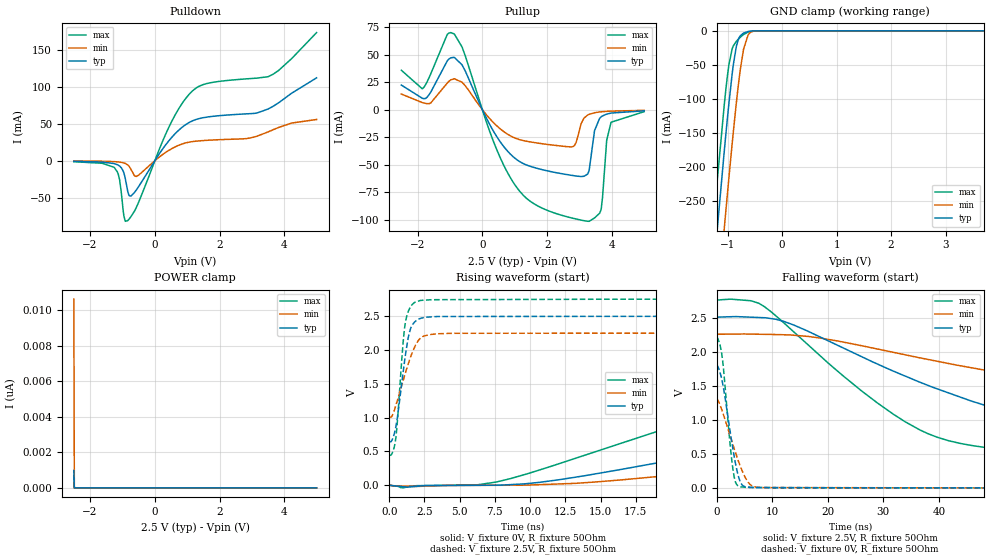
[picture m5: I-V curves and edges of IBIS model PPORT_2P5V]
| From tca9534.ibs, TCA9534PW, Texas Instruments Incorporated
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[Model]   PPORT_2P5V
Model_type   I/O
Polarity   Non-Inverting
Enable   Active-Low
Vinl = .8
Vinh = 2
Vmeas = 1.25
Vref = 2.5
Cref = 15pF
Rref = 50
|   typ   min   max
C_comp   2.511p   2.431p   2.702p
|C_comp (ON state)   2.696p   2.553p   2.895p
|C_comp (OFF state)   2.511p   2.431p   2.702p
[Voltage Range]   2.5   2.25   2.75
[Temperature Range]   27   125   -40
[Pullup Reference]   2.5   2.25   2.75
[Pulldown Reference]   -0   -0   -0
[Power Clamp Reference]   2.5   2.25   2.75
[GND Clamp Reference]   -0   -0   -0
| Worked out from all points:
|   slope of the pulldown table from 0 to 0.375 V, typ, clamps not added: 15.8 ohm
|   slope of the pullup table from 0 to 0.375 V, typ, clamps not added: 17.7 ohm
|   GND clamp passes 1 mA (typ) near -0.62 V on its own axis
|   falling waveform, V_fixture 2.5V, R_fixture 50Ohm: 20-80 % time 36.6ns typ, 66ns min, 21.5ns max; typ from 2.5 V to 0.641 V
|   rising waveform, V_fixture 0V, R_fixture 50Ohm: 20-80 % time 38.7ns typ, 55.5ns min, 23.9ns max; typ from 0 V to 1.78 V
|   rising waveform, V_fixture 2.5V, R_fixture 50Ohm: 20-80 % time 721ps typ, 1.14ns min, 508ps max; typ from 0.641 V to 2.5 V
|   falling waveform, V_fixture 0V, R_fixture 50Ohm: 20-80 % time 2.09ns typ, 3.14ns min, 1.46ns max; typ from 1.78 V to 0 V
[Pulldown]
|   Voltage   I(typ)   I(min)   I(max)
-2.5V     -772.7uA   -289.8uA   -1.301mA
-1.248V   -3.942mA   -1.222mA   -9.315mA
-1.09V    -7.071mA   -1.833mA   -25.27mA
-977.5mV  -13.87mA   -2.72mA    -67.16mA
-917.5mV  -22.81mA   -3.556mA   -81.19mA
-835mV    -41.67mA   -5.666mA   -80.78mA
-572.5mV  -39.52mA   -21.16mA   -63.16mA
410mV     25.73mA    13.43mA    43.16mA
1.085V    52.28mA    25.36mA    90.98mA
1.633V    59.12mA    27.67mA    104.6mA
3.643V    73.35mA    41.76mA    116.6mA
4.992V    112mA      55.73mA    173.1mA
[GND Clamp]
|   Voltage   I(typ)   I(min)   I(max)
-2.5V     -1.557A    -1.668A    -1.488A
-1.278V   -372.4mA   -488.5mA   -299.8mA
-1.21V    -310mA     -425.9mA   -237.7mA
-1.052V   -169.6mA   -283mA     -102mA
-977.5mV  -107.9mA   -217.5mA   -50.54mA
-917.5mV  -64.2mA    -167.1mA   -26.74mA
-842.5mV  -24.2mA    -108.2mA   -15.78mA
-767.5mV  -7.412mA   -57.34mA   -9.428mA
-707.5mV  -3.328mA   -27.12mA   -5.464mA
-617.5mV  -960.2uA   -5.322mA   -1.644mA
-475mV    -67.74uA   -189.6uA   -85.75uA
4.992V    0A         0A         0A
[Pullup]
|   Voltage   I(typ)   I(min)   I(max)
-2.5V     22.39mA    14.21mA    35.9mA
-1.847V   10.34mA    6.416mA    19.11mA
-1.083V   44.38mA    24.22mA    68.51mA
-865mV    47.62mA    28.19mA    68.91mA
1.025V    -44.65mA   -26.02mA   -69.28mA
2.788V    -59.91mA   -33.7mA    -98.78mA
3.147V    -60.51mA   -7.419mA   -101.1mA
3.29V     -55.87mA   -4.304mA   -101.6mA
3.658V    -6.767mA   -1.96mA    -91.58mA
3.837V    -4.033mA   -1.535mA   -27.89mA
3.973V    -3.071mA   -1.319mA   -11.44mA
4.992V    -1.073mA   -633.1uA   -1.823mA
[POWER Clamp]
|   Voltage   I(typ)   I(min)   I(max)
-2.5V     978.3pA    10.63nA    700.4pA
-2.485V   0A         0A         0A
-2.478V   0A         0A         0A
4.992V    0A         0A         0A
[Ramp]
R_load = 50
|   typ   min   max
dV/dt_r   1.06963/3.85271e-08   0.769104/5.55669e-08   1.3173/2.38503e-08
dV/dt_f   1.11552/3.65108e-08   0.746971/6.60089e-08   1.38455/2.14496e-08
[Falling Waveform]
V_fixture = 2.5V
V_fixture_min = 2.25V
V_fixture_max = 2.75V
R_fixture = 50Ohm
C_fixture = 0F
|   Time   V(typ)   V(min)   V(max)
0s        2.5V       2.25V      2.75V
8.572ns   2.497V     2.253V     2.66V
13.86ns   2.39V      2.24V      2.291V
25.89ns   1.933V     2.089V     1.436V
36.63ns   1.549V     1.907V     847.9mV
45.97ns   1.271V     1.761V     620.9mV
59.14ns   983.9mV    1.583V     520.3mV
85.7ns    744.5mV    1.327V     465.3mV
152.3ns   651.6mV    1.077V     446.4mV
499.9ns   640.8mV    1.005V     442.4mV
[Rising Waveform]
V_fixture = 0V
V_fixture_min = 0V
V_fixture_max = 0V
R_fixture = 50Ohm
C_fixture = 0F
|   Time   V(typ)   V(min)   V(max)
0s        1.331uV    48.96nV    1.164uV
7.59ns    1.465mV    34.56uV    47.71mV
12.07ns   82.45mV    20.04mV    320.4mV
25.54ns   573.8mV    263.5mV    1.198V
37.99ns   978.9mV    508mV      1.768V
48.06ns   1.232V     672.8mV    1.994V
64.71ns   1.516V     884.6mV    2.118V
100.7ns   1.718V     1.135V     2.178V
152.3ns   1.769V     1.246V     2.192V
499.9ns   1.783V     1.282V     2.196V
[Rising Waveform]
V_fixture = 2.5V
V_fixture_min = 2.25V
V_fixture_max = 2.75V
R_fixture = 50Ohm
C_fixture = 0F
|   Time   V(typ)   V(min)   V(max)
0s        640.8mV    1.005V     442.4mV
266.4ps   701.2mV    1.054V     502mV
480.5ps   874.2mV    1.186V     715.7mV
988.3ps   1.67V      1.546V     2.11V
1.246ns   2.052V     1.725V     2.5V
1.431ns   2.255V     1.843V     2.605V
1.692ns   2.385V     1.989V     2.682V
2.241ns   2.467V     2.178V     2.731V
2.964ns   2.488V     2.228V     2.741V
499.9ns   2.5V       2.25V      2.75V
[Falling Waveform]
|Gnd
V_fixture = 0V
V_fixture_min = 0V
V_fixture_max = 0V
R_fixture = 50Ohm
C_fixture = 0F
|   Time   V(typ)   V(min)   V(max)
0s        1.783V     1.282V     2.196V
546.8ps   1.707V     1.227V     2.111V
1.039ns   1.546V     1.118V     1.889V
2.491ns   790.6mV    745.6mV    575.2mV
3.139ns   465mV      578.2mV    164.9mV
4.128ns   113.7mV    345.9mV    19.53mV
5.306ns   13.44mV    128.2mV    7.013mV
6.518ns   6.099mV    21.75mV    5.47mV
8.675ns   3.423mV    4.234mV    4.936mV
499.9ns   1.331uV    84.24nV    1.164uV
